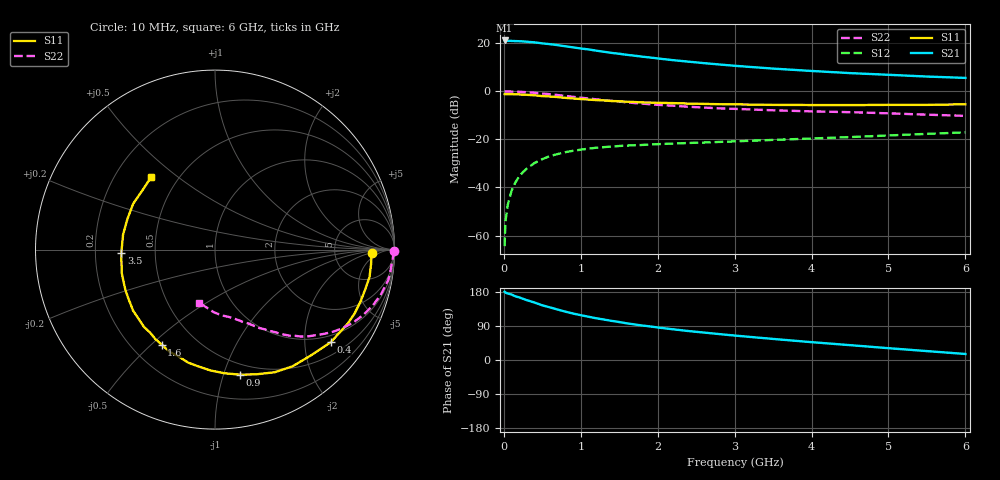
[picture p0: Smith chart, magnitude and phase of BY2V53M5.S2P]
! SIEMENS Small Signal Semiconductors
! BFY420
! Si NPN RF SIEGET Grounded Emitter Transistor in MICRO-X
! VCE = 2.5 V  IC = 3.5 mA
! Common Emitter S-Parameters:  October  1996
# GHz  S  MA  R  50
!  f  S11  S21  S12  S22
! GHz  MAG  ANG  MAG  ANG  MAG  ANG  MAG  ANG
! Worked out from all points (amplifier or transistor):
!   36 points, 10 MHz to 6 GHz, reference 50 ohm
!   highest |S21| = 21.2 dB at 10 MHz (marker M1)
!   |S21| within 3 dB of that: start of sweep to 924.1 MHz
!   unconditionally stable (mu >= 1): 3.481 GHz to end of sweep
!   at 250 MHz: K = 0.09, MSG = 27.2 dB, |S12| = -33.6 dB
!   at 1.4 GHz: K = 0.42, MSG = 19.5 dB, |S12| = -23.0 dB
!   at 6 GHz: K = 1.18, MAG = 8.8 dB, |S12| = -17.1 dB
!   S11 on the Smith chart (normalised r, x): 10 MHz: 15, -2; 400 MHz: 0.81, -2.63; 900 MHz: 0.40, -1.13; 1.6 GHz: 0.32, -0.54; 3.5 GHz: 0.31, -0.02; 6 GHz: 0.35, +0.40
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0.01  0.8756 -1.2  11.44 180.0  0.0006 99.8  0.9946 -0.5
0.02  0.8723 -2.2  11.4 178.0  0.0019 78.8  0.9943 -1.0
0.05  0.8732 -5.2  11.22 175.6  0.0043 87.2  0.9925 -2.5
0.1  0.8744 -10.0  11.2 172.8  0.0085 83.7  0.9869 -5.1
0.15  0.8659 -14.9  11.1 168.0  0.0127 80.9  0.9845 -7.7
0.2  0.8605 -20.0  11.04 165.3  0.017 79.5  0.9797 -10.1
0.25  0.8554 -24.6  10.93 161.4  0.021 76.0  0.9674 -12.6
0.4  0.8259 -38.7  10.44 151.6  0.0323 69.3  0.9324 -19.6
0.5  0.7962 -47.6  9.948 144.3  0.0388 64.5  0.9022 -23.9
0.6  0.7807 -56.4  9.573 138.8  0.045 60.3  0.8706 -27.8
0.7  0.7597 -64.1  9.138 133.1  0.0496 56.7  0.8371 -31.4
0.9  0.7101 -78.8  8.201 122.6  0.058 50.1  0.7689 -37.6
1.1  0.6734 -92.3  7.438 114.2  0.0643 45.2  0.7097 -42.9
1.4  0.6282 -109.0  6.301 103.3  0.0708 39.5  0.6355 -49.0
1.6  0.6067 -119.3  5.746 96.7  0.0743 36.8  0.5907 -52.4
1.8  0.5867 -128.1  5.262 91.0  0.0765 34.6  0.5547 -55.2
2.2  0.569 -143.3  4.454 81.0  0.0819 31.5  0.502 -60.5
2.8  0.5395 -161.1  3.621 68.4  0.0885 29.1  0.4421 -67.0
3.5  0.5224 -178.0  2.972 55.6  0.0976 27.5  0.4032 -73.6
4.5  0.5171 160.6  2.394 39.2  0.1117 24.7  0.3685 -84.1
5.5  0.5222 140.6  2.03 23.5  0.1304 21.0  0.3268 -98.0
6  0.538 131.5  1.903 15.9  0.14 18.7  0.3088 -106.4
